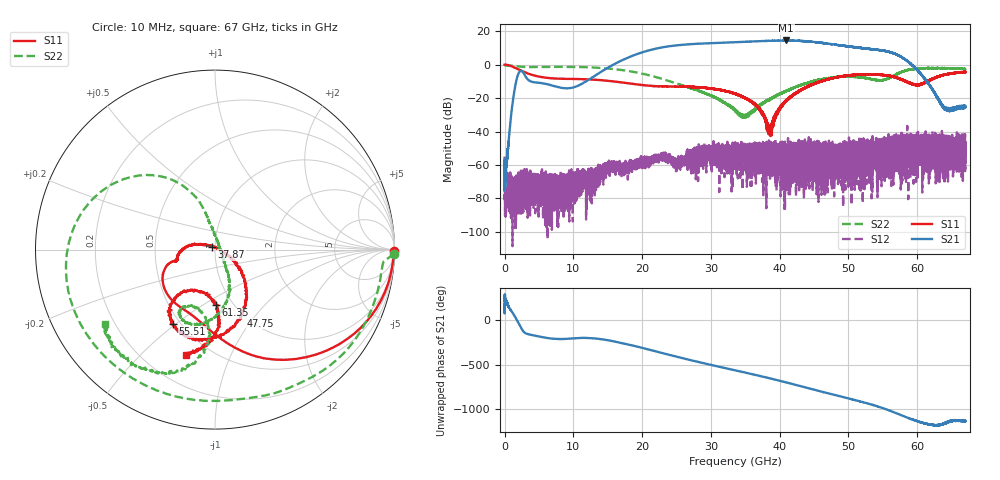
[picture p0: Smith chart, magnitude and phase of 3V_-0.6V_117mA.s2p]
! MARKI MICROWAVE INC.
! Date:  10/21/2020
! Model Number:  AMM-7210CH
! Description:  2-port Small Signal S-parameter data for AMM-7210CH
! Frequency Range:  10 MHz to 67 GHz
! Port Configuration:  PORT 1: Input
!  PORT 2: Output
! Bias Condition: Vd = +3.0V, Vg = -0.6V
! AMM-7210CH s2p files are only valid for small signal conditions (below -10 dBm input power)
# Hz S  dB  R 50
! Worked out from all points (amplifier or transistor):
!   20001 points, 10 MHz to 67 GHz, reference 50 ohm
!   highest |S21| = 14.4 dB at 40.93 GHz (marker M1)
!   |S21| within 3 dB of that: 24.89 GHz to 48.93 GHz (24.04 GHz wide, 65.1 % of centre)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
!   unconditionally stable (mu >= 1): start of sweep to end of sweep
!   at 11.17 GHz: K = 2464.70, MAG = -5.6 dB, |S12| = -74.3 dB
!   at 33.51 GHz: K = 86.85, MAG = 13.5 dB, |S12| = -58.3 dB
!   at 67 GHz: K = 547.90, MAG = -19.9 dB, |S12| = -46.3 dB
!   S11 on the Smith chart (normalised r, x): 10 MHz: open; 37.87 GHz: 0.97, +0.03; 47.75 GHz: 0.98, -0.85; 55.51 GHz: 0.46, -0.49; 61.35 GHz: 0.83, -0.57; 67 GHz: 0.39, -0.68
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1e7  -0.03 -0.5  -59.92 169.1  -54.98 -52.4  -0.01 -1.4
2.22067e9  -3.22 -62.5  -4.01 -60.5  -77.65 -4.9  -1.17 -61.5
1.117723e10  -8.68 -132.9  -11.62 161.9  -68.47 154.1  -1.48 -168.9
1.700201e10  -10.64 -160.0  2.40 105.2  -61.05 116.7  -3.23 149.3
1.990268e10  -12.15 -164.3  7.18 51.7  -55.86 129.1  -5.31 130.3
2.234112e10  -12.98 -163.4  9.81 3.0  -54.74 101.5  -7.86 117.3
2.465562e10  -13.13 -164.3  11.32 -43.3  -56.29 63.9  -10.76 108.7
2.768692e10  -13.45 -169.5  12.36 -101.2  -56.74 62.8  -14.89 102.5
3.08388e10  -14.89 -179.9  12.94 -157.6  -53.98 62.5  -20.13 94.4
3.3505e10  -17.28 169.1  13.37 155.8  -58.35 42.6  -27.00 69.6
3.786605e10  -32.84 140.0  14.10 77.9  -52.03 -80.3  -22.23 -49.8
4.093419e10  -21.48 -24.1  14.43 19.4  -54.56 178.1  -15.80 -61.6
4.268263e10  -16.28 -35.1  14.21 -15.8  -47.35 -113.1  -12.81 -69.9
4.467223e10  -12.04 -47.1  13.70 -56.7  -60.56 7.8  -10.23 -79.8
4.775042e10  -8.07 -68.3  12.11 -118.3  -60.48 77.2  -7.55 -98.0
5.124395e10  -6.04 -93.2  10.27 172.9  -66.63 172.5  -7.35 -116.5
5.368574e10  -5.97 -109.0  9.03 120.8  -52.90 66.3  -8.96 -117.5
5.550787e10  -6.44 -119.5  7.99 73.7  -52.25 154.1  -8.77 -100.2
5.583612e10  -6.66 -121.4  7.68 64.5  -41.64 -88.2  -8.08 -97.8
5.858271e10  -10.32 -128.1  2.11 -19.9  -56.37 -129.4  -3.35 -103.6
6.134939e10  -10.15 -89.4  -9.80 -89.5  -46.87 39.8  -2.15 -122.3
6.7e10  -4.56 -105.6  -25.30 -58.9  -46.33 -4.5  -2.53 -145.8
